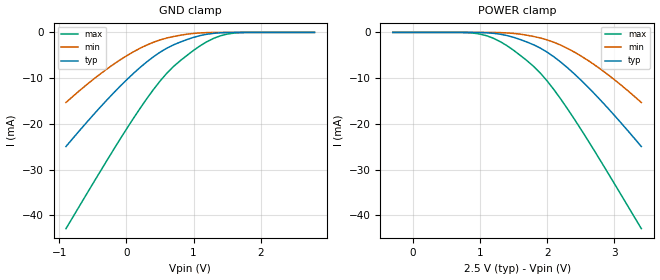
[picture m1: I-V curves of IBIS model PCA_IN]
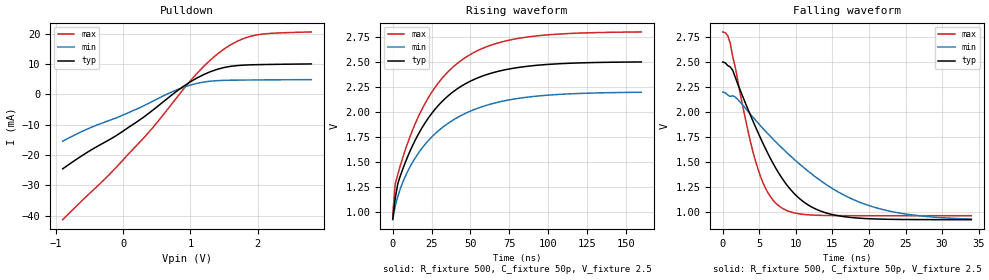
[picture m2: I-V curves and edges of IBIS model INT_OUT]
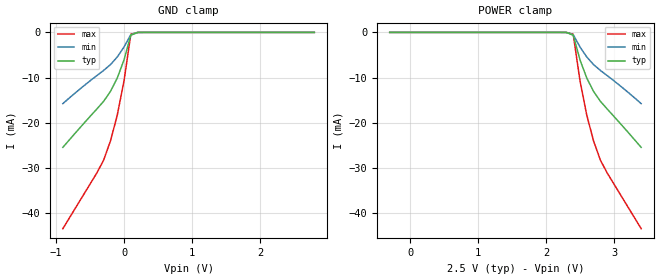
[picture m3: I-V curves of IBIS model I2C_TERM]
|  PCA9541 IBIS MODEL  by NXP Semiconductors, Specialty Logic, Tempe, AZ
|  2-to-1 I2C demultiplexer with interrupt logic and reset
|   Packages: SO16. TSSOP16, HVQFN16
[IBIS Ver]   3.2
[Comment Char]   |_char
| VDD Typ:2.5V, Min:2.2v, Max: 2.8v
[File name]   pca9541_2_5v.ibs
[File Rev]   1.0
[Date]   Apr 11, 2008 11:56:48 AM
[Source]
Generated by Seshadri Venkataramanan using IbisToolKit.
[Notes]
[Disclaimer]
(C) Copyright 2007 NXP Semiconductors
All rights reserved
NXP Semiconductors (NXP) does not warrant that this model and any other
accompanying information (Model) accurately or fully represents the
operating characteristics and specifications of the semiconductor
products to which the Model relates.  Moreover, the Model is furnished
on an "as is" and with "all faults" basis, and without support or
warranty of any kind.  NXP disclaims all warranties, whether expressed
or implied or statutory, including without limitation all implied
warranties of non-infringement, merchantability and fitness for any
purpose, and those arising from a course of dealing or usage of trade.
NXP does not convey any license under its or any third party's patents,
copyrights or other intellectual property or proprietary rights.
You and your company assume any and all risks and liability arising out
of the application or use of the Model.
In no event shall NXP be liable for any direct, indirect, special,
consequential or incidental damages, however caused, whether in
warranty, contract or tort (including negligence), strict liability or
other legal theory, including, without limitation, for lost profits,
business interruption, or corruption or loss of data or information,
arising out of or in connection with the use of or the inability to use
the Model, even if NXP has been advised of the possibility of such
damages.
NXP provides the Model as a courtesy to our customers. You and your
company shall not distribute, convey, sell, or give the Model to anyone
else without receiving prior written permission from NXP.
NXP reserves the right to make changes without notice to the Model to
improve reliability, function, or design.
Please be aware that your receipt and subsequent use of the Model shall
serve as acceptance of these terms and conditions.  If you do not
accept these terms, return or destroy the Model immediately.
[Copyright]
2008
[Component]   pca9541-1D
Si_location Pin
Timing_location Pin
[Manufacturer]   NXP Semiconductors
| [Package]   SO16
| [Package]   SO16
[Package]
|  variable   typ   min   max
R_pkg   1.75E-01   1.28E-01   2.11E-01
L_pkg   5.03E-09   3.94E-09   6.26E-09
C_pkg   0.794E-12   0.715E-12   0.869E-12
[Pin] signal_name   model_name   R_pin   L_pin   C_pin
1   INT0B   INT_OUT   1.99E-01  6.26E-09  0.822E-12
2   SDA_MST0   I2C_TERM   2.11E-01  5.46E-09  0.869E-12
3   SCL_MST0   I2C_TERM   1.56E-01  4.44E-09  0.760E-12
4   RESETB   PCA_IN   1.28E-01  3.94E-09  0.717E-12
5   SCL_MST1   I2C_TERM   1.28E-01  3.94E-09  0.715E-12
6   SDA_MST1   I2C_TERM   1.56E-01  4.44E-09  0.760E-12
7   INT1B   INT_OUT   2.11E-01  5.46E-09  0.869E-12
8   VSS   GND   1.99E-01  6.26E-09  0.843E-12
9   A0   PCA_IN   1.99E-01  6.26E-09  0.843E-12
10   A1   PCA_IN   2.11E-01  5.46E-09  0.869E-12
11   A2   PCA_IN   1.56E-01  4.44E-09  0.760E-12
12   A0(I2C_SEL)   PCA_IN   1.28E-01  3.94E-09  0.717E-12
13   SCL_SLAVE   I2C_TERM   1.28E-01  3.94E-09  0.715E-12
14   SDA_SLAVE   I2C_TERM   1.56E-01  4.44E-09  0.760E-12
15   INT_INB   PCA_IN   2.11E-01  5.46E-09  0.869E-12
16   VDD   POWER   1.99E-01  6.26E-09  0.843E-12
[Series Pin Mapping] pin_2 model_name   function_table_group
2   14   PCA_SW1   1
6   14   PCA_SW1   2
3   13   PCA_SW1   1
5   13   PCA_SW1   2
[Series Switch Groups]
|  1 /
On 1 /
|  2/
On 2 /
[Component]   pca9541-1PW
Si_location Pin
Timing_location Pin
[Manufacturer]   NXP Semiconductors
| [Package]   TSSOP16
| [Package]   TSSOP16
[Package]
| variable   typ   min   max
R_pkg   3.95E-02   3.52E-02   4.56E-02
L_pkg   1.94E-09   1.65E-09   2.40E-09
C_pkg   0.446E-12   0.335E-12   0.771E-12
[Pin] signal_name   model_name   R_pin   L_pin   C_pin
1   INT0B   INT_OUT   3.52E-02  2.40E-09  0.436E-12
2   SDA_MST0   I2C_TERM   3.70E-02  1.93E-09  0.438E-12
3   SCL_MST0   I2C_TERM   4.56E-02  1.76E-09  0.345E-12
4   RESETB   PCA_IN   4.00E-02  1.65E-09  0.335E-12
5   SCL_MST1   I2C_TERM   4.00E-02  1.65E-09  0.335E-12
6   SDA_MST1   I2C_TERM   4.56E-02  1.76E-09  0.345E-12
7   INT1B   INT_OUT   3.70E-02  1.93E-09  0.438E-12
8   VSS   GND   3.52E-02  2.40E-09  0.452E-12
9   A0   PCA_IN   3.52E-02  2.40E-09  0.452E-12
10   A1   PCA_IN   3.70E-02  1.93E-09  0.438E-12
11   A2   PCA_IN   4.56E-02  1.76E-09  0.345E-12
12   A0(I2C_SEL)   PCA_IN   4.00E-02  1.65E-09  0.771E-12
13   SCL_SLAVE   I2C_TERM   4.00E-02  1.65E-09  0.771E-12
14   SDA_SLAVE   I2C_TERM   4.56E-02  1.76E-09  0.345E-12
15   INT_INB   PCA_IN   3.70E-02  1.93E-09  0.438E-12
16   VDD   POWER   3.52E-02  2.40E-09  0.452E-12
[Series Pin Mapping] pin_2 model_name   function_table_group
2   14   PCA_SW1   1
6   14   PCA_SW1   2
3   13   PCA_SW1   1
5   13   PCA_SW1   2
[Series Switch Groups]
|  1 /
On 1 /
|  2/
On 2 /
[Component]   pca9541-1BS
Si_location Pin
Timing_location Pin
[Manufacturer]   NXP Semiconductors
[Package]
|  variable   typ   min   max
R_pkg   403m   325m   479m
L_pkg   112nh   98nh   127nh
C_pkg   0.142p   0.129p   0.157p
[Package Model]   hvqfn16
[Pin] signal_name   model_name
1   SCL_MST0   I2C_TERM
2   RESETB   PCA_IN
3   SCL_MST1   I2C_TERM
4   SDA_MST1   I2C_TERM
5   INT1B   INT_OUT
6   VSS   GND
7   A0   PCA_IN
8   A1   PCA_IN
9   A2   PCA_IN
10   A0(I2C_SEL)   PCA_IN
11   SCL_SLAVE   I2C_TERM
12   SDA_SLAVE   I2C_TERM
13   INT_INB   PCA_IN
14   VDD   POWER
15   INT0B   INT_OUT
16   SDA_MST0   I2C_TERM
[Series Pin Mapping] pin_2 model_name   function_table_group
16   12   PCA_SW1   1
4   12   PCA_SW1   2
1   11   PCA_SW1   1
3   11   PCA_SW1   2
[Series Switch Groups]
|  1 /
On 1 /
|  2/
On 2 /
[Define Package Model]   hvqfn16
[Manufacturer]   Unknown
[OEM]   Unknown
[Description]   none
[Number of Pins]   16
[Pin Numbers]
|   1 =
1
|   2 =
2
|   3 =
3
|   4 =
4
|   5 =
5
|   6 =
6
|   7 =
7
|   8 =
8
|   9 =
9
|   10 =
10
|   11 =
11
|   12 =
12
|   13 =
13
|   14 =
14
|   15 =
15
|   16 =
16
[Model Data]
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[End Model Data]
[End Package Model]
[Model]   PCA_SW1
Model_type Series_switch
C_comp   5.5p   5.3p   5.7p
[Temperature Range] 27   85   -40
[Voltage Range]   2.5   2.2   2.8
[On]
[R Series]   12   4   24
[L Series]   0   0   0
[C Series]   2p   1p   5p
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[Off]
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| Models and submodels in the file (4): PCA_IN (Input), INT_OUT (Open_drain), I2C_TERM (Terminator), PCA_SW1 (Series_switch)
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[Model]   PCA_IN
Model_type Input
Vinh=2.1
Vinl=0.9
C_comp   2.44p   2.2p   2.6p
[Temperature Range] 27   85   -40
[Voltage Range]   2.5   2.2   2.8
[GND Clamp]
-900mV    -24.97mA   -15.34mA   -42.94mA
-400mV    -16.54mA   -9.212mA   -30.68mA
100mV     -9.042mA   -4.284mA   -18.91mA
300mV     -6.496mA   -2.789mA   -14.58mA
500mV     -4.347mA   -1.652mA   -10.67mA
600mV     -3.467mA   -1.234mA   -8.962mA
800mV     -2.129mA   -624.7uA   -6.214mA
1V        -1.085mA   -223.8uA   -3.935mA
1.2V      -397.7uA   -48.08uA   -2.026mA
1.5V      -30.06uA   -1.319uA   -369.3uA
1.8V      -376.8nA   -17.99nA   -10.01uA
2.8V      11.35pA    120.5pA    22.32fA
[POWER Clamp]
-300mV    11.35pA    120.5pA    22.32fA
700mV     -376.8nA   -17.99nA   -10.01uA
1V        -30.06uA   -1.319uA   -369.3uA
1.3V      -397.7uA   -48.08uA   -2.026mA
1.5V      -1.085mA   -223.8uA   -3.935mA
1.7V      -2.129mA   -624.7uA   -6.214mA
1.9V      -3.467mA   -1.234mA   -8.962mA
2V        -4.347mA   -1.652mA   -10.67mA
2.2V      -6.496mA   -2.789mA   -14.58mA
2.4V      -9.042mA   -4.284mA   -18.91mA
2.9V      -16.54mA   -9.212mA   -30.68mA
3.4V      -24.97mA   -15.34mA   -42.94mA
[Model]   INT_OUT
Model_type Open_drain
Vref=2.5
Vmeas=1.25
Rref=500
Cref=50p
C_comp   2.44p   2.2p   2.6p
[Model Spec]
Vmeas   1.65   1.485   1.815
[Temperature Range] 27   85   -40
[Voltage Range]   2.5   2.2   2.8
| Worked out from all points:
|   slope of the pulldown table from 0 to 0.375 V, typ, clamps not added: 65.2 ohm
|   falling waveform, R_fixture 500, C_fixture 50p, V_fixture 2.5: 20-80 % time 6.55ns typ, 12.1ns min, 3.55ns max; typ from 2.5 V to 0.928 V
|   rising waveform, R_fixture 500, C_fixture 50p, V_fixture 2.5: 20-80 % time 34.8ns typ, 37.6ns min, 35.2ns max; typ from 0.928 V to 2.5 V
[Pulldown]
-900mV    -24.53mA   -15.4mA    -41.31mA
-500mV    -18.61mA   -11.08mA   -32.65mA
-100mV    -13.53mA   -7.685mA   -23.98mA
400mV     -5.89mA    -2.692mA   -12mA
800mV     1.134mA    1.562mA    -959.9uA
1.1V      5.466mA    3.673mA    7.006mA
1.4V      8.302mA    4.569mA    13.31mA
1.6V      9.292mA    4.709mA    16.41mA
1.7V      9.548mA    4.74mA     17.6mA
1.9V      9.782mA    4.782mA    19.23mA
2.2V      9.919mA    4.828mA    20.17mA
2.8V      10.08mA    4.901mA    20.63mA
[Falling Waveform]
R_fixture=500
C_fixture=50p
V_fixture=2.5
V_fixture_min=2.2
V_fixture_max=2.8
0s        2.5V       2.2V       2.8V
1.03ns    2.451V     2.157V     2.687V
3.434ns   2.032V     2.01V      1.821V
4.808ns   1.801V     1.894V     1.436V
6.182ns   1.588V     1.785V     1.197V
7.899ns   1.365V     1.658V     1.054V
10.99ns   1.11V      1.453V     981.2mV
15.11ns   977mV      1.234V     968.7mV
22.67ns   931.8mV    1.016V     967.6mV
34ns      927.8mV    934mV      967.6mV
[Rising Waveform]
R_fixture=500
C_fixture=50p
V_fixture=2.5
V_fixture_min=2.2
V_fixture_max=2.8
0s        927.8mV    921.3mV    967.6mV
1.616ns   1.134V     1.055V     1.279V
3.232ns   1.279V     1.151V     1.371V
4.848ns   1.357V     1.229V     1.459V
14.55ns   1.718V     1.54V      1.883V
27.47ns   2.03V      1.784V     2.249V
43.64ns   2.251V     1.96V      2.509V
59.8ns    2.368V     2.062V     2.646V
82.42ns   2.447V     2.138V     2.738V
160ns     2.498V     2.195V     2.798V
[Ramp]
R_load=500
dV/dt_r   9.416E-1/2.212E-9   9.055E-1/1.825E-9   9.301E-1/1.908E-9
dV/dt_f   9.432E-1/9.289E-10   9.077E-1/6.438E-10   9.322E-1/3.208E-10
|[End   INT_OUT
| [End   SDAX,SCLX
[Model]   I2C_TERM
Model_type Terminator
C_comp   5.5p   5.3p   5.7p
[Temperature Range] 27   85   -40
[Voltage Range]   2.5   2.2   2.8
[GND Clamp]
-900mV    -25.45mA   -15.76mA   -43.44mA
-400mV    -16.96mA   -9.558mA   -31.11mA
-300mV    -15.26mA   -8.419mA   -28.28mA
-200mV    -13.08mA   -7.138mA   -24.06mA
-100mV    -10.12mA   -5.451mA   -18.36mA
0V        -6.088mA   -3.228mA   -10.74mA
100mV     -620.3uA   -506.3uA   -422.9uA
200mV     -14.95uA   -24.09uA   -3.091uA
2.8V      160.4pA    185.8pA    156.9pA
[POWER Clamp]
-300mV    160.4pA    185.8pA    156.9pA
2.3V      -14.95uA   -24.09uA   -3.091uA
2.4V      -620.3uA   -506.3uA   -422.9uA
2.5V      -6.088mA   -3.228mA   -10.74mA
2.6V      -10.12mA   -5.451mA   -18.36mA
2.7V      -13.08mA   -7.138mA   -24.06mA
2.8V      -15.26mA   -8.419mA   -28.28mA
2.9V      -16.96mA   -9.558mA   -31.11mA
3.4V      -25.45mA   -15.76mA   -43.44mA
